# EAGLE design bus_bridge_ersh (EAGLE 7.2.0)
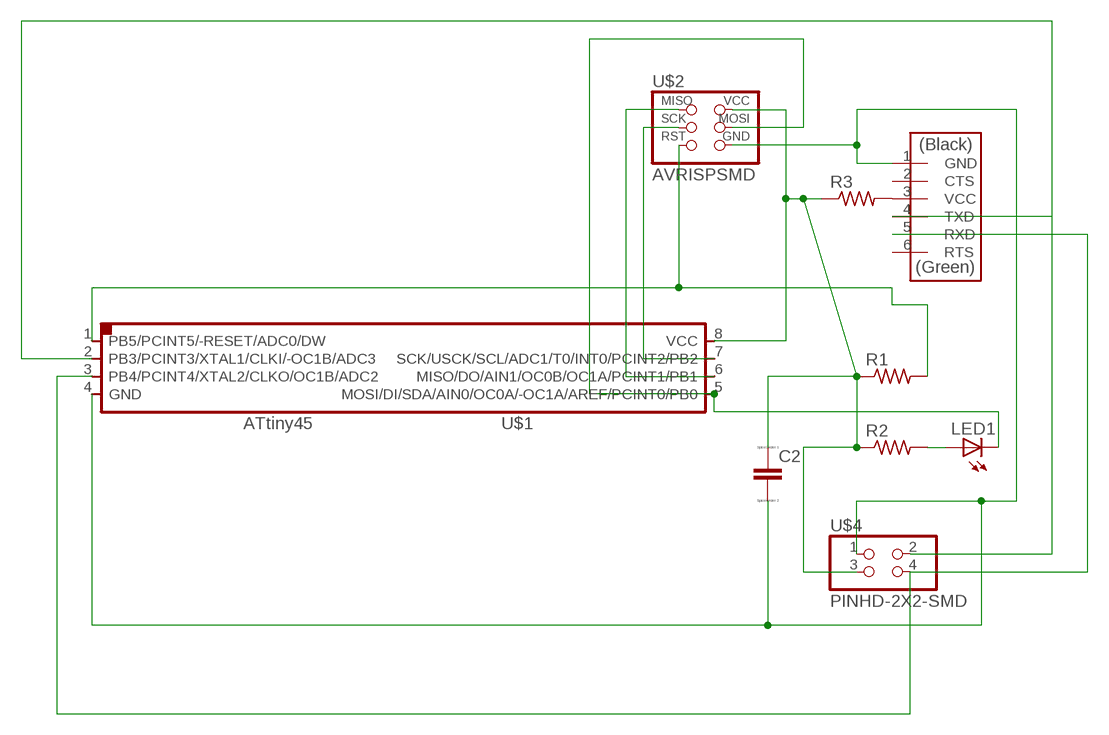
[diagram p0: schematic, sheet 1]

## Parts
C2  CC1206  [C1206]
LED1  LEDKA-3528ASYC  [KA-3528ASYC]
R1  RES-US1206  [R1206]
R2  RES-US1206  [R1206]
R3  RES-US1206  [R1206]
U$1  ATTINY45SI  [SOIC8]
U$2  AVRISPSMD  [2X03SMD]
U$3  FTDI-SMD-HEADER  [1X06SMD]
U$4  PINHD-2X2-SMD  [2X02SMD]

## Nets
N$1: C2.1 R1.1 R2.1 R3.1 U$1.8(VCC) U$2.2(VCC) U$4.3
N$2: C2.2 U$1.4(GND) U$2.6(GND) U$3.1(GND) U$4.1
N$3: R1.2 U$1.1(PB5/PCINT5/-RESET/ADC0/DW) U$2.5(RST)
N$4: LED1.A R2.2
N$5: LED1.C U$1.5(MOSI/DI/SDA/AIN0/OC0A/-OC1A/AREF/PCINT0/PB0) U$2.4(MOSI)
N$6: U$1.6(MISO/DO/AIN1/OC0B/OC1A/PCINT1/PB1) U$2.1(MISO)
N$7: U$1.7(SCK/USCK/SCL/ADC1/T0/INT0/PCINT2/PB2) U$2.3(SCK)
N$8: U$1.2(PB3/PCINT3/XTAL1/CLKI/-OC1B/ADC3) U$3.4(TXD) U$4.2
N$9: U$1.3(PB4/PCINT4/XTAL2/CLKO/OC1B/ADC2) U$3.5(RXD) U$4.4
N$10: R3.2 U$3.3(VCC)
Unconnected: U$3.2(CTS) U$3.6(RTS)

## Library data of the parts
C2 = eagle-ltspice:C: CAPACITOR, European symbol; SPICEMODEL: NONE; SPICEPREFIX: C
LED1 = led:LED: LED
R1-R3 = fab:RES-US: Resistor (US Symbol)
U$1 = fab:ATTINY45
U$2 = fab:AVRISP
U$3 = fab:FTDI-SMD-HEADER
U$4 = fab:PINHD-2X2-SMD

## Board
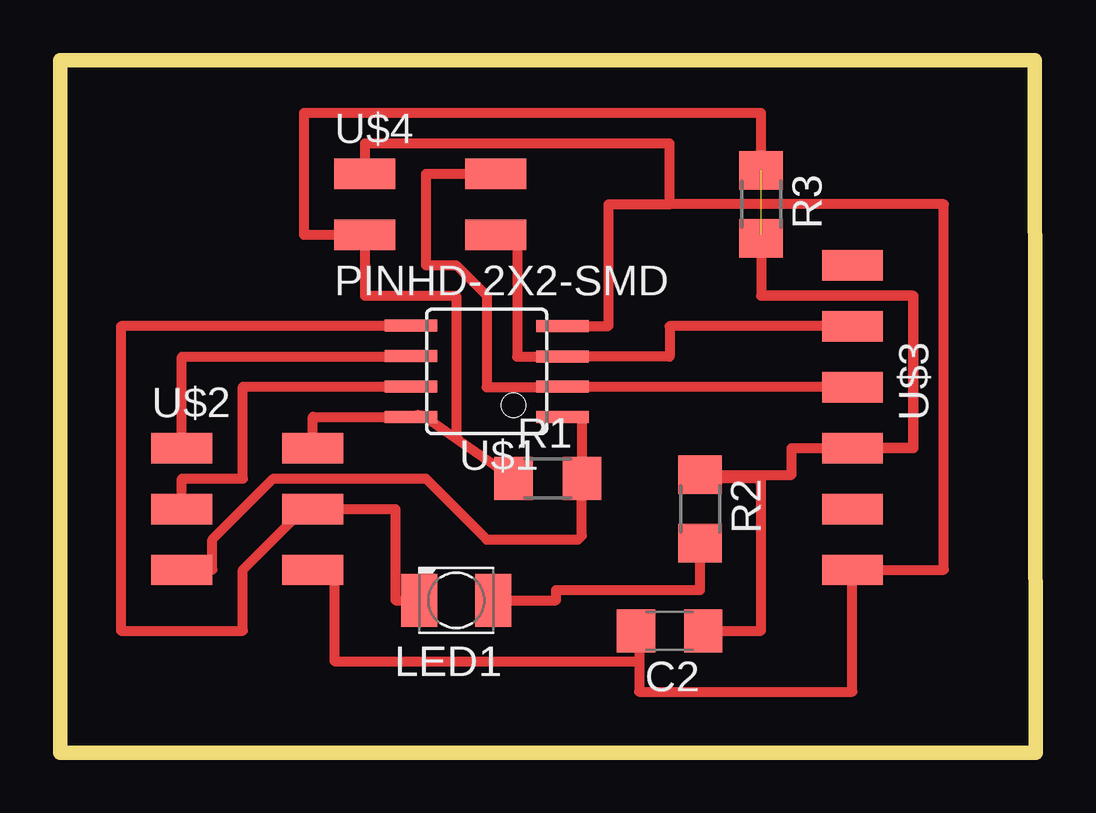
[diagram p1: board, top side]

Size 40.66 x 28.88 mm. Coordinates in mm from the lower left corner, seen from the top.
Outline: 0,0 40.66,0 40.62,28.88 0,28.88 0,0
Copper layers (1*16): Top 0.035mm / dielectric 1.5mm / Bottom 0.035mm
Design rules "default": minimum track width 10mil, minimum drill 24mil, track to track 8mil, track to pad 8mil, pad to pad 8mil, via to via 8mil, smd to smd 8mil, copper to edge 40mil, drill to drill 8mil, minimum pad ring 10mil, minimum via ring 8mil, stop-mask expansion 4mil, vias tented up to drill 0mil, thermal gap 10mil

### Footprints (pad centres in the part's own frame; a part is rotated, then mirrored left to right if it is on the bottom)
C1206 = smd 1.6 x 1.8: 1 -1.4,0; 2 1.4,0
KA-3528ASYC = smd 1.5 x 2.2: A -1.55,0; C 1.55,0
R1206 = smd 1.6 x 1.803: 1 -1.422,0; 2 1.422,0
SOIC8 = smd 0.5 x 2.2: 1 -1.905,-3.154; 2 -0.645,-3.154; 3 0.625,-3.154; 4 1.895,-3.154; 5 1.905,3.154; 6 0.635,3.154; 7 -0.635,3.154; 8 -1.905,3.154
2X03SMD = smd 2.54 x 1.27: 1 -2.54,2.54; 2 2.92,2.54; 3 -2.54,0; 4 2.92,0; 5 -2.54,-2.54; 6 2.92,-2.54
1X06SMD = smd 2.54 x 1.27: 1 0,6.35; 2 0,3.81; 3 0,1.27; 4 0,-1.27; 5 0,-3.81; 6 0,-6.35
2X02SMD = smd 2.54 x 1.27: 1 -2.54,1.27; 2 2.92,1.27; 3 -2.54,-1.27; 4 2.92,-1.27

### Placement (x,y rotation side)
C2  25.4,5.08 180 top
LED1  16.51,6.35 180 top
R1  20.32,11.43 0 top
R2  26.67,10.16 270 top
R3  29.21,22.86 270 top
U$1  17.78,15.9 90 top
U$2  7.62,10.16 0 top
U$3  33.02,13.97 180 top
U$4  15.24,22.86 0 top

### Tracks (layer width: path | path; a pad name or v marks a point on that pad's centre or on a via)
N$1  (1 unrouted)
  Top 0.406: U$2.2 10.54,14 U$1.8 arc-65 15.24,13.97 16.69,12.96 | R1.1 16.69,12.96 | C2.1 29.21,5.08 29.21,11.43 26.67,11.43 R2.1 30.48,11.58 30.48,12.7 35.56,12.7 35.56,19.05 29.21,19.05 29.21,21.59 | R3.1 29.21,26.67 10.16,26.67 10.16,21.59 U$4.3 12.7,19.05 16.51,19.05 16.51,13.14 16.69,12.96
N$2
  Top 0.254: U$2.6 11.43,7.62 | C2.2 24.13,5.08
  Top 0.406: 25.4,22.86 36.83,22.86 36.83,7.62 U$3.1 33.02,2.54 24.13,2.54 24.13,3.81 | 25.4,22.86 25.4,25.4 12.7,25.4 U$4.1 | U$1.4 22.86,17.79 22.86,22.86 25.4,22.86 | 11.43,7.62 11.43,3.81 24.13,3.81 | 24.13,5.08 24.13,3.81
N$3
  Top 0.406: U$2.5 6.35,7.62 6.35,8.89 8.89,11.43 15.24,11.43 17.78,8.89 21.59,8.89 21.74,9.04 R1.2 21.74,14 U$1.1
N$4
  Top 0.406: LED1.A 20.68,6.35 20.68,6.78 26.67,6.78 R2.2
N$5
  Top 0.254: U$1.5 14.63,17.78 | 10.16,10.16 U$2.4 | 15.24,6.35 LED1.C
  Top 0.406: 14.63,17.78 2.54,17.78 2.54,5.08 7.62,5.08 7.62,7.62 10.16,10.16 | U$2.4 13.97,10.16 13.97,6.35 LED1.C
N$6
  Top 0.254: 14.63,16.51 U$1.6
  Top 0.406: U$2.1 5.08,16.51 14.63,16.51
N$7
  Top 0.406: U$2.3 5.08,11.43 7.62,11.43 7.62,15.27 U$1.7
N$8
  Top 0.254: 20.93,15.24 U$1.2
  Top 0.406: U$3.4 20.93,15.24 17.78,15.24 17.78,19.05 16.51,20.32 15.24,20.32 15.24,24.13 U$4.2
N$9
  Top 0.254: U$4.4 19.05,21.59 | 20.93,16.51 U$1.3
  Top 0.406: U$3.5 25.4,17.78 25.4,16.51 20.93,16.51 19.05,16.51 19.05,21.59
N$10
  Top 0.406: R3.2 29.21,19.05 35.56,19.05 35.56,12.7 U$3.3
